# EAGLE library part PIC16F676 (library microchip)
14-Pin, Flash-Based 8-Bit CMOS Microcontroller High Performance RISC CPU: * Only 35 instructions to learn - All single-cycle instructions except branches * Operating speed: - DC - 20 MHz oscillator/clock input - DC - 200 ns instruction cycle * Internal and external oscillator options - Precision Internal 4 MHz oscillator factory calibrated to ±1% - External Oscillator support for crystals and resonators - 5?s wake-up from SLEEP, 3.0V, typical * Power saving SLEEP mode * Wide operating voltage range - 2.0V to 5.5V * Industrial and Extended temperature range * Low power Power-on Reset (POR) * Power-up Timer (PWRT) and Oscillator Start-up Timer (OST) * Brown-out Detect (BOD) * Watchdog Timer (WDT) with independent oscillator for reliable operation * Multiplexed MCLR/Input-pin * Interrupt-on-pin change * Individual programmable weak pull-ups * Programmable code protection * High Endurance FLASH/EEPROM Cell - 100,000 write FLASH endurance - 1,000,000 write EEPROM endurance - FLASH/Data EEPROM Retention: > 40 years * Standby Current: - 1 nA @ 2.0V, typical * Operating Current: - 8.5?A @ 32 kHz, 2.0V, typical - 100?A @ 1 MHz, 2.0V, typical * Watchdog Timer Current - 300 nA @ 2.0V, typical * Timer1 oscillator current: - 4?A @ 32 kHz, 2.0V, typical * 12 I/O pins with individual direction control * High current sink/source for direct LED drive * Analog-to-Digital Converter module (PIC16F676): - 10-bit resolution - Programmable 8-channel input - Voltage reference input * In-Circuit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
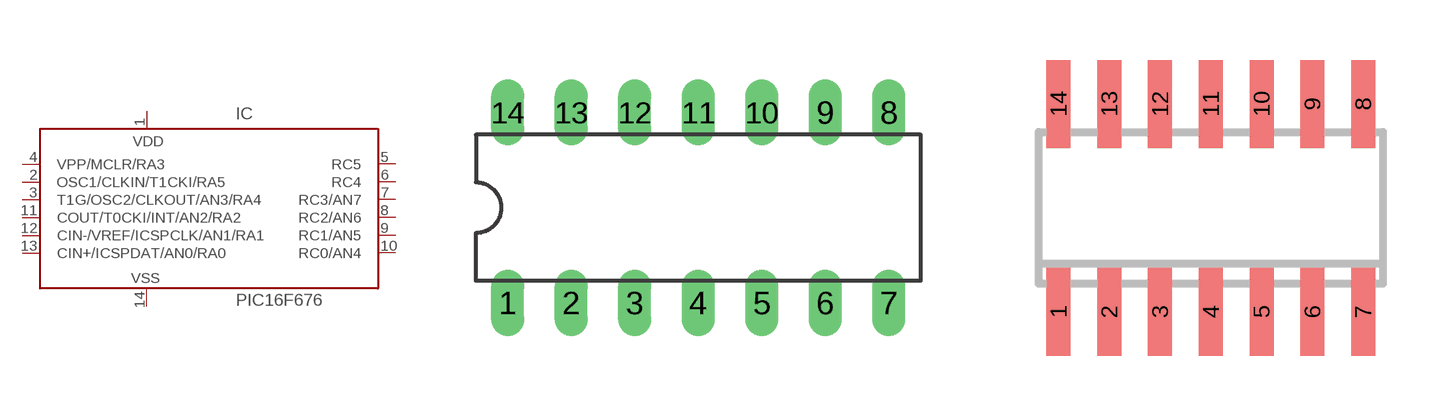
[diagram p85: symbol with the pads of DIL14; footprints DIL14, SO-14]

Designator prefix IC

## PIC16F676P (MF: MICROCHIP; MPN: PIC16F676-I/P; OC_FARNELL: 9760512; OC_NEWARK: 54K2829)  [DIL14]
1  VDD  pwr
2  OSC1/CLKIN/T1CKI/RA5
3  T1G/OSC2/CLKOUT/AN3/RA4
4  VPP/MCLR/RA3  in
5  RC5
6  RC4
7  RC3/AN7
8  RC2/AN6
9  RC1/AN5
10  RC0/AN4
11  COUT/T0CKI/INT/AN2/RA2
12  CIN-/VREF/ICSPCLK/AN1/RA1
13  CIN+/ICSPDAT/AN0/RA0
14  VSS  pwr

## PIC16F676SL (MF: MICROCHIP; MPN: PIC16F676-I/SL; OC_FARNELL: 9760520; OC_NEWARK: 92C4557)  [SO-14]
Pads as for DIL14

## PIC16F676TS (MF: MICROCHIP; MPN: PIC16F676-E/ST; OC_FARNELL: 9760539; OC_NEWARK: 92C4552)  [TSSOP14]
Pads as for DIL14

## Footprint DIL14 (pad centres in mm)
Dual In Line Package
drill 0.813 long: 1 -7.62,-3.81; 2 -5.08,-3.81; 3 -2.54,-3.81; 4 0,-3.81; 5 2.54,-3.81; 6 5.08,-3.81; 7 7.62,-3.81; 8 7.62,3.81; 9 5.08,3.81; 10 2.54,3.81; 11 0,3.81; 12 -2.54,3.81; 13 -5.08,3.81; 14 -7.62,3.81

## Footprint SO-14 (pad centres in mm)
Small Outline Narrow Plastic Gull Wing 150-mil body, package type SL
smd 0.6 x 2.2: 1 -3.81,-2.6; 2 -2.54,-2.6; 3 -1.27,-2.6; 4 0,-2.6; 5 1.27,-2.6; 6 2.54,-2.6; 7 3.81,-2.6; 8 3.81,2.6; 9 2.54,2.6; 10 1.27,2.6; 11 0,2.6; 12 -1.27,2.6; 13 -2.54,2.6; 14 -3.81,2.6

## Footprint TSSOP14 (pad centres in mm)
14-Lead Plastic Thin Shrink Small Outline (ST) - 4.4 mm Body TSSOP Source: http://ww1.microchip.com/downloads/en/DeviceDoc/40039E.pdf
smd 0.35 x 1: 1 -1.95,-2.825; 2 -1.3,-2.825; 3 -0.65,-2.825; 4 0,-2.825; 5 0.65,-2.825; 6 1.3,-2.825; 7 1.95,-2.825; 8 1.95,2.825; 9 1.3,2.825; 10 0.65,2.825; 11 0,2.825; 12 -0.65,2.825; 13 -1.3,2.825; 14 -1.95,2.825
